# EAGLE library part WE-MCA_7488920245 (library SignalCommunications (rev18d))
Multilayer Chip Antenna Characteristics SMD Multilayer Chip Antenna Extremely low profile Very light component Power capacity: 5 W max. Omni-directional Operating temperature: –40 °C to +85 °C High gain Applications applications WLAN Home RF (868 MHz) Bluetooth applications GSM 900 ISM 868/2400 Details see: http://katalog.we-online.de/en/pbs/WE-MCA? Updated by Dan Xu 2014-07-08 2014 (C) Wurth Elektronik
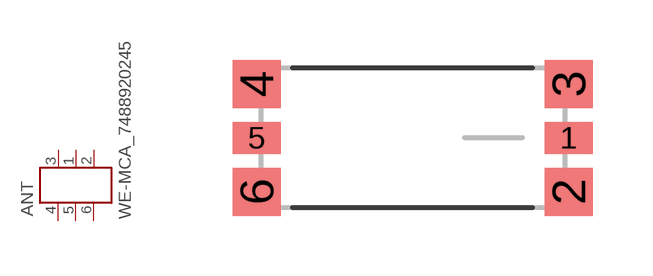
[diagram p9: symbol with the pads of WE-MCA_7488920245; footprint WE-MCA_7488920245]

Designator prefix ANT

## WE-MCA_7488920245  [WE-MCA_7488920245]
1  FP  nc
2  GND1  nc
3  GND2  nc
4  NC1  pwr
5  NC2  pas
6  NC3  pwr

## Footprint WE-MCA_7488920245 (pad centres in mm)
Multiplayer Chip Antenna WE-MCA
smd 1.2 x 0.8: 1 3.9,0; 5 -3.9,0
smd 1.2 x 1.2: 2 3.9,-1.35; 3 3.9,1.35; 4 -3.9,1.35; 6 -3.9,-1.35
